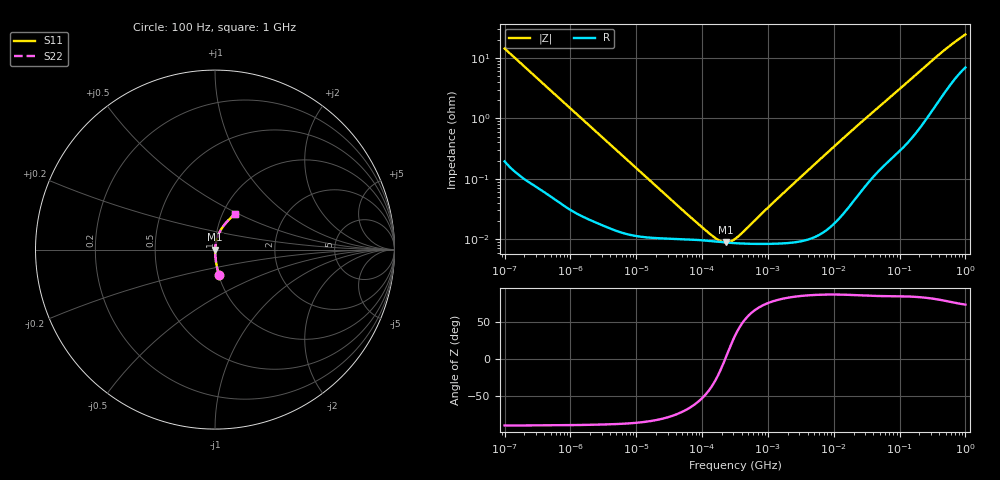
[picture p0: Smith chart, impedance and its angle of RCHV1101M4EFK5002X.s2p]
! RCHV1101M4EFK5002X  S-PARAMETER MODEL  (AEC-Q200 qualified)
! Model Generated by ELNA Corporation (http://www.ty-top.com)
! Version 1.0
! ELNA Control No. 240229
! Copyright (c) 2024 ELNA CO.,LTD. All Rights Reserved.
! Products Name : CONDUCTIVE POLYMER HYBRID ALUMINUM ELECTROLYTIC CAPACITORS
! Characteristics :
!  Capacitance  :  100uF  ,  Rated voltage  :  63V
!  Operating Temp. Range  :  -55 to +105 degC  ,  Endurance  :  5000hr at 105 degC
!  Dimension D  :  10mm  ,  Dimension L  :  12.5mm
! Frequency Range : 100Hz - 1GHz
! External Node Assignments :
!  1  o---| |---o  2
# MHz S RI R 50
!Freq[MHz].  S11 Real  S11 Imag  S21 Real  S21 Imag  S12 Real  S12 Imag  S22 Real  S22 Imag
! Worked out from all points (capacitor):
!   401 points, 100 Hz to 1 GHz, reference 50 ohm
!   read as one part in series: C = 110 uF near 108 Hz
!   lowest |Z| = 8.79 mohm at 229.1 kHz (marker M1)
!   series resonance near 223.7 kHz, so ESL is about 4.6 nH
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0.0001  0.0221 -0.1405  0.9779 0.1405  0.9779 0.1405  0.0221 -0.1405
0.000113  0.0176 -0.1252  0.9824 0.1252  0.9824 0.1252  0.0176 -0.1252
0.000183  0.00721 -0.0782  0.9928 0.0782  0.9928 0.0782  0.00721 -0.0782
0.000309  0.00291 -0.0467  0.9971 0.0467  0.9971 0.0467  0.00291 -0.0467
0.001488  0.000337 -0.00987  0.9997 0.00987  0.9997 0.00987  0.000337 -0.00987
0.022131  0.000104 -0.000672  0.9999 0.000672  0.9999 0.000672  0.000104 -0.000672
0.071203  9.81e-05 -0.000194  0.9999 0.000194  0.9999 0.000194  9.81e-05 -0.000194
0.147062  9.2e-05 -6.16e-05  0.9999 6.16e-05  0.9999 6.16e-05  9.2e-05 -6.16e-05
0.172783  9.04e-05 -3.76e-05  0.9999 3.76e-05  0.9999 3.76e-05  9.04e-05 -3.76e-05
0.229087  8.79e-05 3.5e-06  0.9999 -3.5e-06  0.9999 -3.5e-06  8.79e-05 3.5e-06
0.291743  8.61e-05 3.98e-05  0.9999 -3.98e-05  0.9999 -3.98e-05  8.61e-05 3.98e-05
0.316228  8.56e-05 5.25e-05  0.9999 -5.25e-05  0.9999 -5.25e-05  8.56e-05 5.25e-05
0.342768  8.52e-05 6.56e-05  0.9999 -6.56e-05  0.9999 -6.56e-05  8.52e-05 6.56e-05
0.402717  8.45e-05 9.32e-05  0.9999 -9.32e-05  0.9999 -9.32e-05  8.45e-05 9.32e-05
1.148154  8.37e-05 0.000374  0.9999 -0.000374  0.9999 -0.000374  8.37e-05 0.000374
4.704354  0.000106 0.00159  0.9999 -0.00159  0.9999 -0.00159  0.000106 0.00159
20.06781  0.000472 0.00668  0.9995 -0.00668  0.9995 -0.00668  0.000472 0.00668
69.9842  0.00246 0.0217  0.9975 -0.0217  0.9975 -0.0217  0.00246 0.0217
176.8072  0.0084 0.052  0.9916 -0.052  0.9916 -0.052  0.0084 0.052
395.8221  0.0309 0.1067  0.9691 -0.1067  0.9691 -0.1067  0.0309 0.1067
668.3439  0.0673 0.1562  0.9327 -0.1562  0.9327 -0.1562  0.0673 0.1562
1000  0.1087 0.1965  0.8913 -0.1965  0.8913 -0.1965  0.1087 0.1965
